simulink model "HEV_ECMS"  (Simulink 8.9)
settings: Solver=FixedStepDiscrete  StartTime=0.0  StopTime=400  FixedStep=data.dt  RelTol=1e-3  EnableMultiTasking=on
InitFcn:
  | init_HEV_ECMS
StopFcn:
  | if t(end)==str2num(get_param(char(bdroot(gcb)),'StopTime'))
  | msgbox('Simulation completed')
  | else
  | msgbox('Simulation aborted due to limitation in one of the components','','error')
  | end
undefined symbols (not defined in the file or in its folder): DiscIntNeverNeededParam, Hlhv, I_max, parallelhybrid_ECMS, Q_0, R_i, rho_f, SOC_0, U_oc
libraries: qss_tb_library x3, simulink x2

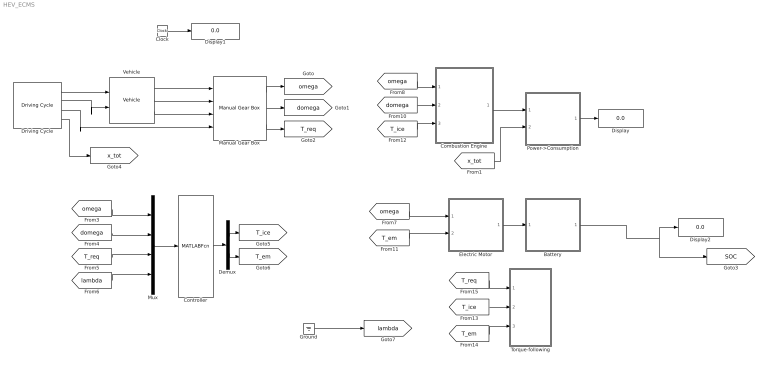
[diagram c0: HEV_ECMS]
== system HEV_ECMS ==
  Battery : Subsystem
  Clock : Clock
  Combustion Engine : Subsystem
  Controller : MATLABFcn  MATLABFcn=parallelhybrid_ECMS(u)
  Demux : Demux  Outputs=2
  Display : Display
  Display1 : Display
  Display2 : Display
  Driving Cycle : qss_tb_library/Driving Cycle/Driving Cycle  Tag=cycle  cyclenr=Europe: EUDC manual  stepsize=1  autostop=on
  Electric Motor : Subsystem
  Ground : Ground
  Manual Gear Box : qss_tb_library/Gear System/Manual Gear Box  Tag=transmission  i_1=15.174  i_2=8.338  i_3=5.378  i_4=3.937  i_5=2.748  i_diff=1  e_GT=0.98  P_GT0=300  w_wheel_min=1
  Mux : Mux
  Power->Consumption : Subsystem
  Torque-following : Subsystem
  Vehicle : qss_tb_library/Vehicle/Vehicle  Tag=vehicle  m_f=750  mt2m_f=5  A_f=1.8  r_wheel=0.3  cw=0.22  mu=0.008
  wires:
  Power->Consumption/1(Consumption) -> Display/1
  Combustion Engine/1(P_f) -> Power->Consumption/1(P_f)
  Driving Cycle/1 -> Vehicle/1
  Driving Cycle/2 -> Vehicle/2
  Driving Cycle/3 -> Manual Gear Box/4
  Vehicle/1 -> Manual Gear Box/1
  Vehicle/2 -> Manual Gear Box/2
  Vehicle/3 -> Manual Gear Box/3
  Clock/1 -> Display1/1
  Manual Gear Box/1 -> [omega]
  Manual Gear Box/2 -> [domega]
  Manual Gear Box/3 -> [T_req]
  [x_tot] -> Power->Consumption/2(x_tot)
  Electric Motor/1(P_em_el) -> Battery/1(P_batt)
  Mux/1 -> Controller/1
  [lambda] -> Mux/4
  [omega] -> Electric Motor/1(w_em)
  [omega] -> Combustion Engine/1(w_gear)
  [domega] -> Combustion Engine/2(dw_gear)
  Controller/1 -> Demux/1
  Demux/1 -> [T_ice]
  [T_em] -> Electric Motor/2(T_em)
  [T_ice] -> Combustion Engine/3(T_gear)
  Driving Cycle/4 -> [x_tot]
  Battery/1(SOC1) -> Display2/1, [SOC]
  [T_ice] -> Torque-following/2("T_ice ")
  [T_em] -> Torque-following/3(T_em)
  [T_req] -> Torque-following/1(T_req)
  Demux/2 -> [T_em]
  [omega] -> Mux/1
  [domega] -> Mux/2
  [T_req] -> Mux/3
  Ground/1 -> [lambda]

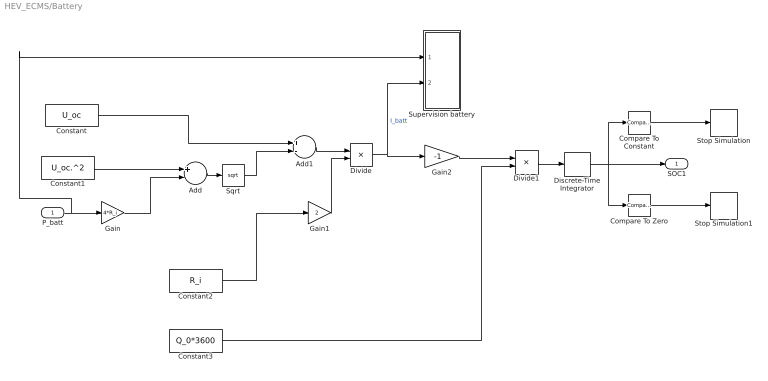
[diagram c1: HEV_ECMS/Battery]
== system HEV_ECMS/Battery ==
  P_batt : Inport
  Add : Sum  Inputs=+-
  Add1 : Sum  Inputs=+-
  Compare To Constant : simulink/Logic and Bit Operations/Compare To Constant  relop=>  const=1  OutDataTypeStr=boolean
  Compare To Zero : simulink/Logic and Bit Operations/Compare To Zero  relop=<  OutDataTypeStr=boolean
  Constant : Constant  Value=U_oc
  Constant1 : Constant  Value=U_oc.^2
  Constant2 : Constant  Value=R_i
  Constant3 : Constant  Value=Q_0*3600
  Discrete-Time Integrator : DiscreteIntegrator  InitialCondition=SOC_0  SampleTime=-1  ICPrevOutput=DiscIntNeverNeededParam  ICPrevScaledInput=DiscIntNeverNeededParam
  Divide : Product  Inputs=*/
  Divide1 : Product  Inputs=*/
  Gain : Gain  Gain=4*R_i
  Gain1 : Gain  Gain=2
  Gain2 : Gain  Gain=-1
  Sqrt : Sqrt
  Stop Simulation : Stop
  Stop Simulation1 : Stop
  Supervision battery : Subsystem  AncestorBlock=qss_tb_library/Energy Buffer/Battery/Battery voltage/Supervision battery
  SOC1 : Outport
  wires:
  P_batt/1 -> Gain/1, Supervision battery/1(P_batt)
  Constant1/1 -> Add/1
  Gain/1 -> Add/2
  Add/1 -> Sqrt/1
  Divide/1 -> Supervision battery/2(I_batt), Gain2/1  "I_batt"
  Divide1/1 -> Discrete-Time Integrator/1
  Sqrt/1 -> Add1/2
  Constant/1 -> Add1/1
  Add1/1 -> Divide/1
  Constant2/1 -> Gain1/1
  Gain1/1 -> Divide/2
  Constant3/1 -> Divide1/2
  Gain2/1 -> Divide1/1
  Discrete-Time Integrator/1 -> Compare To Zero/1, SOC1/1, Compare To Constant/1
  Compare To Zero/1 -> Stop Simulation1/1
  Compare To Constant/1 -> Stop Simulation/1

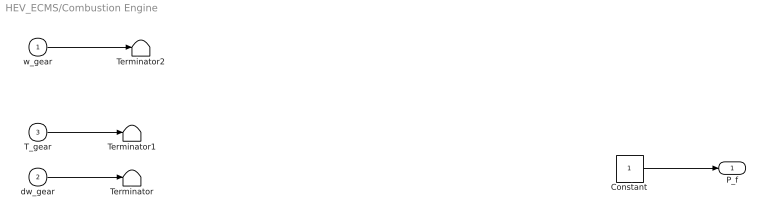
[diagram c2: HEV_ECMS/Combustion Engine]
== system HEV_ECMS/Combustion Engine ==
  w_gear : Inport
  dw_gear : Inport  Port=2
  T_gear : Inport  Port=3
  Constant : Constant
  Terminator : Terminator
  Terminator1 : Terminator
  Terminator2 : Terminator
  P_f : Outport
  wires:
  dw_gear/1 -> Terminator/1
  Constant/1 -> P_f/1
  T_gear/1 -> Terminator1/1
  w_gear/1 -> Terminator2/1

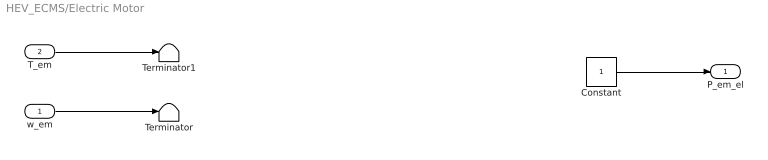
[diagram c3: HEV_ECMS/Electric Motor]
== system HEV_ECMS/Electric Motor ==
  w_em : Inport
  T_em : Inport  Port=2
  Constant : Constant
  Terminator : Terminator
  Terminator1 : Terminator
  P_em_el : Outport
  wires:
  w_em/1 -> Terminator/1
  T_em/1 -> Terminator1/1
  Constant/1 -> P_em_el/1

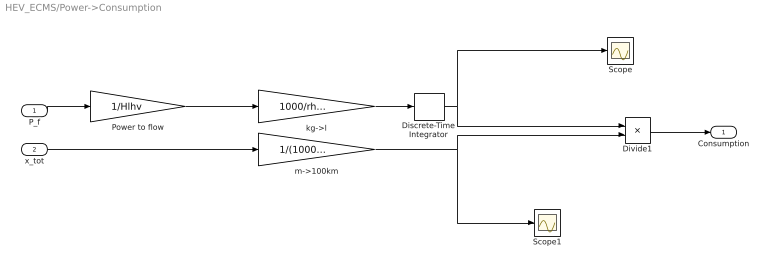
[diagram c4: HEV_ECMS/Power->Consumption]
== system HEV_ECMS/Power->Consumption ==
  P_f : Inport
  x_tot : Inport  Port=2
  Discrete-Time Integrator : DiscreteIntegrator  IntegratorMethod=Integration: Trapezoidal  SampleTime=-1  ICPrevOutput=DiscIntNeverNeededParam  ICPrevScaledInput=DiscIntNeverNeededParam
  Divide1 : Product  Inputs=*/
  Power to flow : Gain  Gain=1/Hlhv
  Scope : Scope
  Scope1 : Scope
  kg->l : Gain  Gain=1000/rho_f
  m->100km : Gain  Gain=1/(100000)
  Consumption : Outport
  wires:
  Divide1/1 -> Consumption/1
  P_f/1 -> Power to flow/1
  Power to flow/1 -> kg->l/1
  kg->l/1 -> Discrete-Time Integrator/1
  x_tot/1 -> m->100km/1
  m->100km/1 -> Divide1/2, Scope1/1
  Discrete-Time Integrator/1 -> Divide1/1, Scope/1

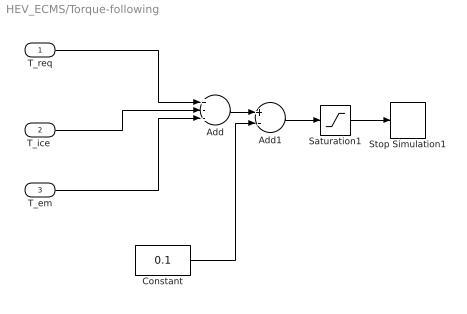
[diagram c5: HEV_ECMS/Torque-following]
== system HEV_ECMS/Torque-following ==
  T_req : Inport
  "T_ice " : Inport  Port=2
  T_em : Inport  Port=3
  Add : Sum  Inputs=+--
  Add1 : Sum  Inputs=+-
  Constant : Constant  Value=0.1
  Saturation1 : Saturate  UpperLimit=inf  LowerLimit=0
  Stop Simulation1 : Stop
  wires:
  "T_ice "/1 -> Add/2
  T_em/1 -> Add/3
  T_req/1 -> Add/1
  Saturation1/1 -> Stop Simulation1/1
  Add/1 -> Add1/1
  Constant/1 -> Add1/2
  Add1/1 -> Saturation1/1

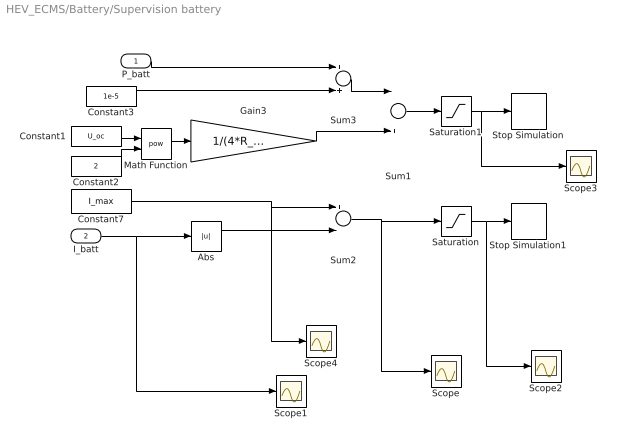
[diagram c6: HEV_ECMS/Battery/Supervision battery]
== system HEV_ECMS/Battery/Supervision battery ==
  P_batt : Inport
  I_batt : Inport  Port=2
  Abs : Abs
  Constant1 : Constant  Value=U_oc
  Constant2 : Constant  Value=2
  Constant3 : Constant  Value=1e-5
  Constant7 : Constant  Value=I_max
  Gain3 : Gain  Gain=1/(4*R_i)
  Math Function : Math  Operator=pow
  Saturation : Saturate  UpperLimit=0  LowerLimit=-inf
  Saturation1 : Saturate  UpperLimit=0  LowerLimit=-inf
  Scope{,1..4} (5 alike) : Scope
  Stop Simulation : Stop
  Stop Simulation1 : Stop
  Sum1 : Sum  Inputs=-+
  Sum2 : Sum  Inputs=+-
  Sum3 : Sum
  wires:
  Abs/1 -> Sum2/2
  I_batt/1 -> Abs/1, Scope1/1
  Sum2/1 -> Saturation/1, Scope/1
  Constant7/1 -> Sum2/1, Scope4/1
  P_batt/1 -> Sum3/1
  Sum1/1 -> Saturation1/1
  Saturation1/1 -> Stop Simulation/1, Scope3/1
  Saturation/1 -> Stop Simulation1/1, Scope2/1
  Gain3/1 -> Sum1/2
  Sum3/1 -> Sum1/1
  Constant1/1 -> Math Function/1
  Math Function/1 -> Gain3/1
  Constant2/1 -> Math Function/2
  Constant3/1 -> Sum3/2
